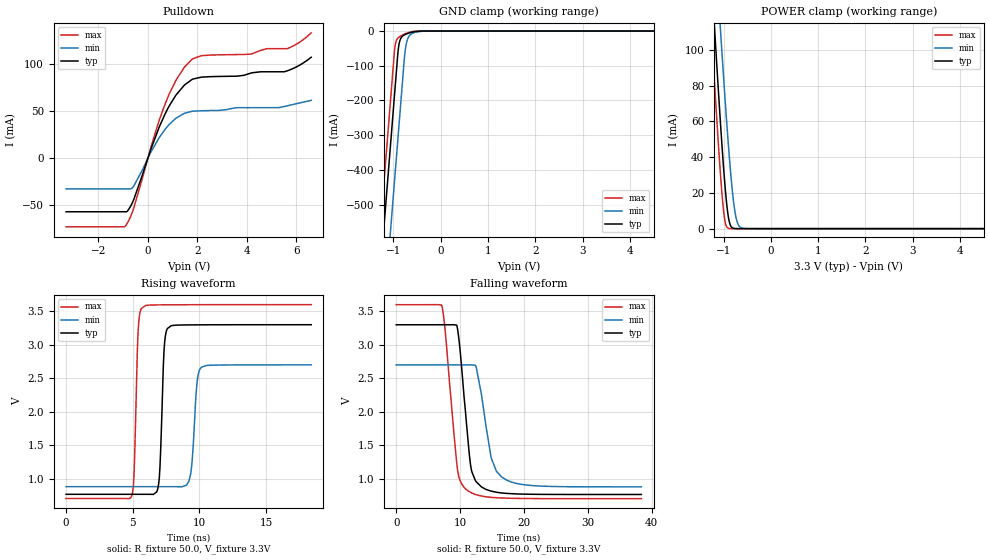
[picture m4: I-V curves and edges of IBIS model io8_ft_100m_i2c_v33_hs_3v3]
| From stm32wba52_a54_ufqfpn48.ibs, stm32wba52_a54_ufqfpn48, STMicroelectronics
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[Model]   io8_ft_100m_i2c_v33_hs_3v3
Model_type I/O_open_drain
Polarity   Non-Inverting
Enable   Active-Low
| CAP_THRESHOLD on pad IOFT is "UDTCAPC" :
| Rising=30.0% of vddiom   Falling=70.0% of vddiom
| C_comp min and max val. don't necessarily correlate with the min and max pvt
| but are the smallest and greatest pad capacitance found.
| var   typ   min   max
C_comp   2.70452pF  2.60096pF  2.73919pF
|C_comp_pulldown   2.70452pF  2.60096pF  2.73919pF
Vinl = 1.35V
Vinh = 1.8V
Vmeas = 1.65V   | Reference voltage for timing measurements
Cref  = 50.0pF   | Timing specification test load capacitance value
Rref  = 1.0MOhm   | Timing specification test load resistance value
Vref  = 1.815V   | Timing specification test load voltage
[Model Spec]
| TIME_THRESHOLD on pin ZII2CV11 is "CMOS" :
| Rising=50.0% of vdd   Falling=50.0% of vdd
Vinl 1.28450V 1.07650V 1.38450V
Vinh 1.79550V 1.49050V 1.94250V
| variable   typ   min   max
[Temperature Range] 25.0 140.0 -40.0
| variable   typ   min   max
[Voltage Range] 3.3V 2.7V 3.6V
| variable   typ   min   max
[POWER Clamp Reference] 3.3V 2.7V 3.6V
| variable   typ   min   max
[GND Clamp Reference] 0V 0V 0V
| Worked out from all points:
|   slope of the pulldown table from 0 to 0.495 V, typ, clamps not added: 14 ohm
|   GND clamp passes 1 mA (typ) near -0.51 V on its own axis
|   POWER clamp passes 1 mA (typ) near -0.83 V on its own axis
|   rising waveform, R_fixture 50.0, V_fixture 3.3V: 20-80 % time 256ps typ, 332ps min, 231ps max; typ from 0.764 V to 3.3 V
|   falling waveform, R_fixture 50.0, V_fixture 3.3V: 20-80 % time 1.43ns typ, 1.96ns min, 1.58ns max; typ from 3.3 V to 0.764 V
[POWER Clamp]
-3.3V     1.123A     1.139A     1.091A
-1.36V    189.2mA    238.8mA    158.1mA
-1.25V    139mA      190.3mA    108.1mA
-1.18V    107.9mA    159.9mA    77.22mA
-1.06V    57.23mA    109.3mA    28.68mA
-980mV    27.6mA     77.28mA    5.935mA
-900mV    6.895mA    47.74mA    242.8uA
-820mV    594.6uA    22.85mA    5.912uA
-760mV    69.41uA    9.714mA    358.6nA
-700mV    7.83uA     2.919mA    21.86nA
-630mV    611.5nA    529.9uA    954.5pA
6.6V      0A         0A         0A
[GND Clamp]
-3.3V     -4.134A    -4.382A    -4.006A
-1.59V    -1.227A    -1.475A    -1.099A
-1.25V    -648.9mA   -896.7mA   -520.9mA
-980mV    -189.9mA   -437.7mA   -61.92mA
-970mV    -172.9mA   -420.7mA   -48.45mA
-910mV    -70.86mA   -318.7mA   -21.03mA
-880mV    -37.23mA   -267.7mA   -17.31mA
-750mV    -9.908mA   -55.25mA   -7.768mA
-710mV    -7.626mA   -27.41mA   -5.608mA
-650mV    -4.885mA   -11.6mA    -3.058mA
-360mV    -31.22uA   -443.6uA   -1.188uA
6.6V      2.31nA     2.655uA    974.6pA
| variable   typ   min   max
[Pullup Reference] 3.3V 2.7V 3.6V
| variable   typ   min   max
[Pulldown Reference] 0V 0V 0V
[Pulldown]
-3.3V     -56.7mA    -32.4mA    -72.73mA
-890mV    -56.7mA    -32.4mA    -71.32mA
-570mV    -43.94mA   -29.54mA   -52.99mA
120mV     9.474mA    6.407mA    11.48mA
700mV     47.33mA    30.97mA    57.88mA
1.14V     67.41mA    42.74mA    83.2mA
1.78V     83.75mA    50.04mA    105.1mA
2.17V     86.37mA    50.65mA    109.1mA
4.16V     90.61mA    53.89mA    110.8mA
4.82V     92.03mA    53.89mA    116.6mA
5.63V     93.04mA    55.89mA    116.6mA
6.6V      107.5mA    61.71mA    133.4mA
[Ramp]
dV/dt_r 1.5215V/251.30544ps 1.09298V/330.66045ps 1.73919V/226.73429ps
dV/dt_f 1.52157V/1.42663ns 1.09309V/1.84531ns 1.73924V/1.57597ns
R_load = 50.0
| Removed startup time: 0s 0s 0s  .
| Removed end time: 18.4ns.
[Rising Waveform]
R_fixture   = 50.0
V_fixture   = 3.3V
V_fixture_min = 2.7V
V_fixture_max = 3.6V
0s        764mV      878.1mV    701.3mV
4.9ns     764mV      878.1mV    727.6mV
5.1ns     764mV      878.1mV    1.055V
5.4ns     764.1mV    878.1mV    3.177V
5.65ns    764mV      878.1mV    3.544V
6.95ns    922.7mV    878.1mV    3.597V
7.6ns     3.243V     878.1mV    3.598V
9.25ns    3.297V     983.2mV    3.599V
10.15ns   3.298V     2.664V     3.599V
18.4ns    3.3V       2.7V       3.6V
| Removed startup time: 0s 0s 0s  .
| Removed end time: 38.4ns.
[Falling Waveform]
R_fixture   = 50.0
V_fixture   = 3.3V
V_fixture_min = 2.7V
V_fixture_max = 3.6V
0s        3.3V       2.7V       3.6V
7.15ns    3.3V       2.7V       3.585V
7.65ns    3.3V       2.7V       3.23V
9.55ns    3.268V     2.7V       1.177V
11ns      1.834V     2.7V       836.7mV
11.65ns   1.203V     2.7V       794.9mV
12.4ns    973.1mV    2.694V     764.4mV
14.9ns    813.2mV    1.305V     721.2mV
16.5ns    787mV      1.027V     711.7mV
38.4ns    764.1mV    878.2mV    701.3mV
